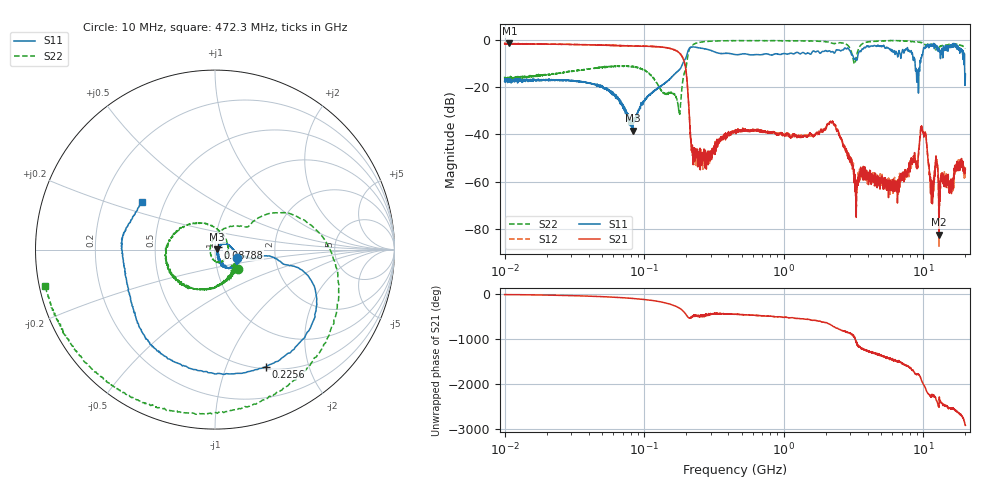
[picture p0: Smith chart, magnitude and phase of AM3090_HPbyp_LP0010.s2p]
# Hz S DB R 50
!freq MagS11 AngS11 MagS21 AngS21 MagS12 AngS12 MagS22 AngS22
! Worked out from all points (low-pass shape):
!   3201 points, 10 MHz to 20 GHz, reference 50 ohm
!   highest |S21| = -1.40 dB at 10.82 MHz (marker M1); lowest = -82.5 dB at 12.95 GHz (marker M2)
!   |S21| within 3 dB of the highest: start of sweep to 166.9 MHz; 167.1283 MHz to 167.4294 MHz (301.1 kHz wide, 0.18 % of centre)
!   lowest |S11| = -38.4 dB at 82.62 MHz (marker M3), VSWR 1.02, Z = 51.2 + j0.0753 ohm
!   |S11| at or under -10 dB: start of sweep to 188.9 MHz; 8.726 GHz to 9.45 GHz (724.6 MHz wide, 7.97 % of centre); 19.73 GHz to end of sweep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
!   |S22| runs from -31.5 to -0.2 dB; largest |S21 - S12| = 0.044
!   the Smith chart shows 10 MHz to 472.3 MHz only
!   S11 on the Smith chart (normalised r, x): 10 MHz: 1.28, -0.12; 87.88 MHz: 1.03, +0.03; 225.6 MHz: 0.53, -1.39; 472.3 MHz: 0.37, +0.26
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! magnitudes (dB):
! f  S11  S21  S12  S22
! 10 MHz  -17.5  -1.7  -1.6  -15.5
! 10.82 MHz  -17.6  -1.4  -1.6  -17.8
! 35.55 MHz  -17.7  -2.0  -2.0  -12.8
! 82.62 MHz  -38.4  -2.6  -2.5  -11.3
! 87.88 MHz  -33.5  -2.6  -2.6  -11.5
! 126.1 MHz  -20.5  -2.9  -2.8  -19.3
! 176.7 MHz  -12.9  -5.3  -5.2  -29.7
! 191.1 MHz  -9.3  -8.2  -8.2  -15.6
! 225.6 MHz  -3.0  -47.5  -49.7  -1.9
! 447.2 MHz  -6.2  -38.6  -39.0  -0.3
! 472.3 MHz  -6.2  -38.6  -38.4  -0.3
! 1.59 GHz  -5.3  -40.3  -40.3  -0.4
! 2.228 GHz  -4.9  -34.4  -34.5  -1.4
! 3.281 GHz  -7.9  -61.4  -64.0  -8.4
! 5.639 GHz  -3.6  -60.1  -58.4  -0.3
! 9.068 GHz  -14.6  -53.1  -52.6  -0.9
! 9.901 GHz  -5.3  -38.7  -38.5  -1.3
! 11.44 GHz  -2.6  -69.0  -62.1  -1.9
! 12.29 GHz  -3.0  -49.6  -51.1  -4.1
! 12.95 GHz  -3.4  -82.5  -87.3  -3.1
! 17.14 GHz  -2.4  -55.2  -54.6  -1.8
! 20 GHz  -14.5  -54.8  -53.9  -3.6
